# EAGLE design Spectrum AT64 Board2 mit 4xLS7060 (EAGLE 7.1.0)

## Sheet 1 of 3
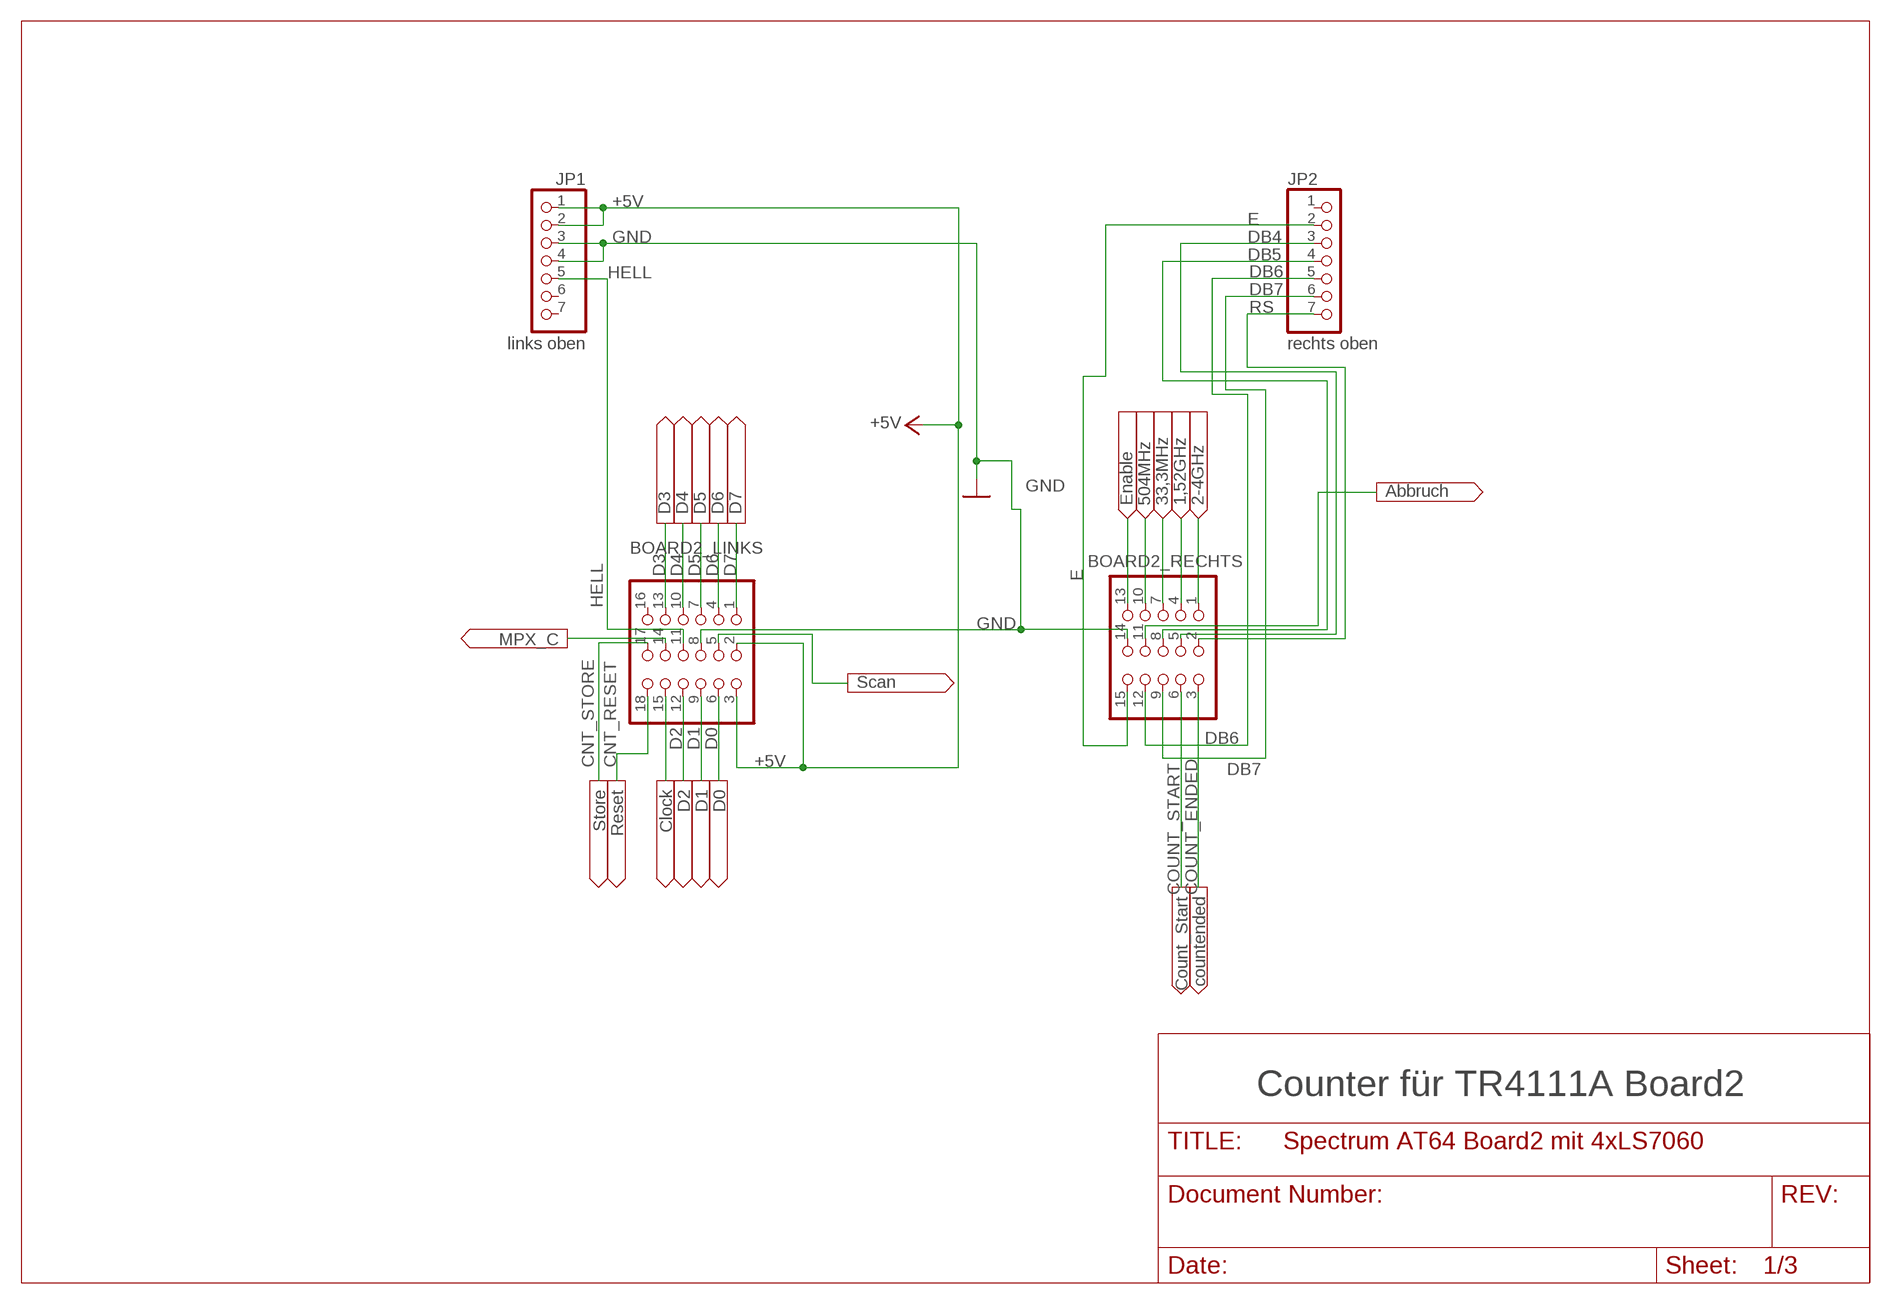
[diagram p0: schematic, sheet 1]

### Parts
BOARD2_LINKS  links  3X06  [3X06]
BOARD2_RECHTS  rechts  PINHEAD3X05  [3X05]
JP1  links oben  PINHD-1X7  [1X07]
JP2  rechts oben  PINHD-1X7  [1X07]

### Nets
1,52GHZ: BOARD2_RECHTS.4 ; also sheet 3
2-4GHZ: BOARD2_RECHTS.1 ; also sheet 3
33,3MHZ: BOARD2_RECHTS.7 ; also sheet 3
504MHZ: BOARD2_RECHTS.10 ; also sheet 3
+5V: BOARD2_LINKS.2 BOARD2_LINKS.3 JP1.1 JP1.2 ; also sheet 2,3
ABBRUCH: BOARD2_RECHTS.11 ; also sheet 2
CLOCK: BOARD2_LINKS.15 ; also sheet 2
CNT_RESET: BOARD2_LINKS.18 ; also sheet 3
CNT_STORE: BOARD2_LINKS.17 ; also sheet 3
COUNT_ENDED: BOARD2_RECHTS.3 ; also sheet 2
COUNT_START: BOARD2_RECHTS.6 ; also sheet 2
D0: BOARD2_LINKS.6 ; also sheet 3
D1: BOARD2_LINKS.9 ; also sheet 3
D2: BOARD2_LINKS.12 ; also sheet 3
D3: BOARD2_LINKS.13 ; also sheet 3
D4: BOARD2_LINKS.10 ; also sheet 3
D5: BOARD2_LINKS.7 ; also sheet 3
D6: BOARD2_LINKS.4 ; also sheet 3
D7: BOARD2_LINKS.1 ; also sheet 3
DB4: BOARD2_RECHTS.5 JP2.3
DB5: BOARD2_RECHTS.8 JP2.4
DB6: BOARD2_RECHTS.12 JP2.5
DB7: BOARD2_RECHTS.9 JP2.6
E: BOARD2_RECHTS.15 JP2.2
ENABLE: BOARD2_RECHTS.13 ; also sheet 3
GND: BOARD2_LINKS.8 BOARD2_RECHTS.14 JP1.3 JP1.4 ; also sheet 2,3
HELL: BOARD2_LINKS.11 JP1.5
MPX_C: BOARD2_LINKS.14 ; also sheet 2
RS: BOARD2_RECHTS.2 JP2.7
SCAN: BOARD2_LINKS.5 ; also sheet 3
Unconnected: BOARD2_LINKS.16 JP1.6 JP1.7 JP2.1

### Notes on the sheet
- Counter für TR4111A Board2

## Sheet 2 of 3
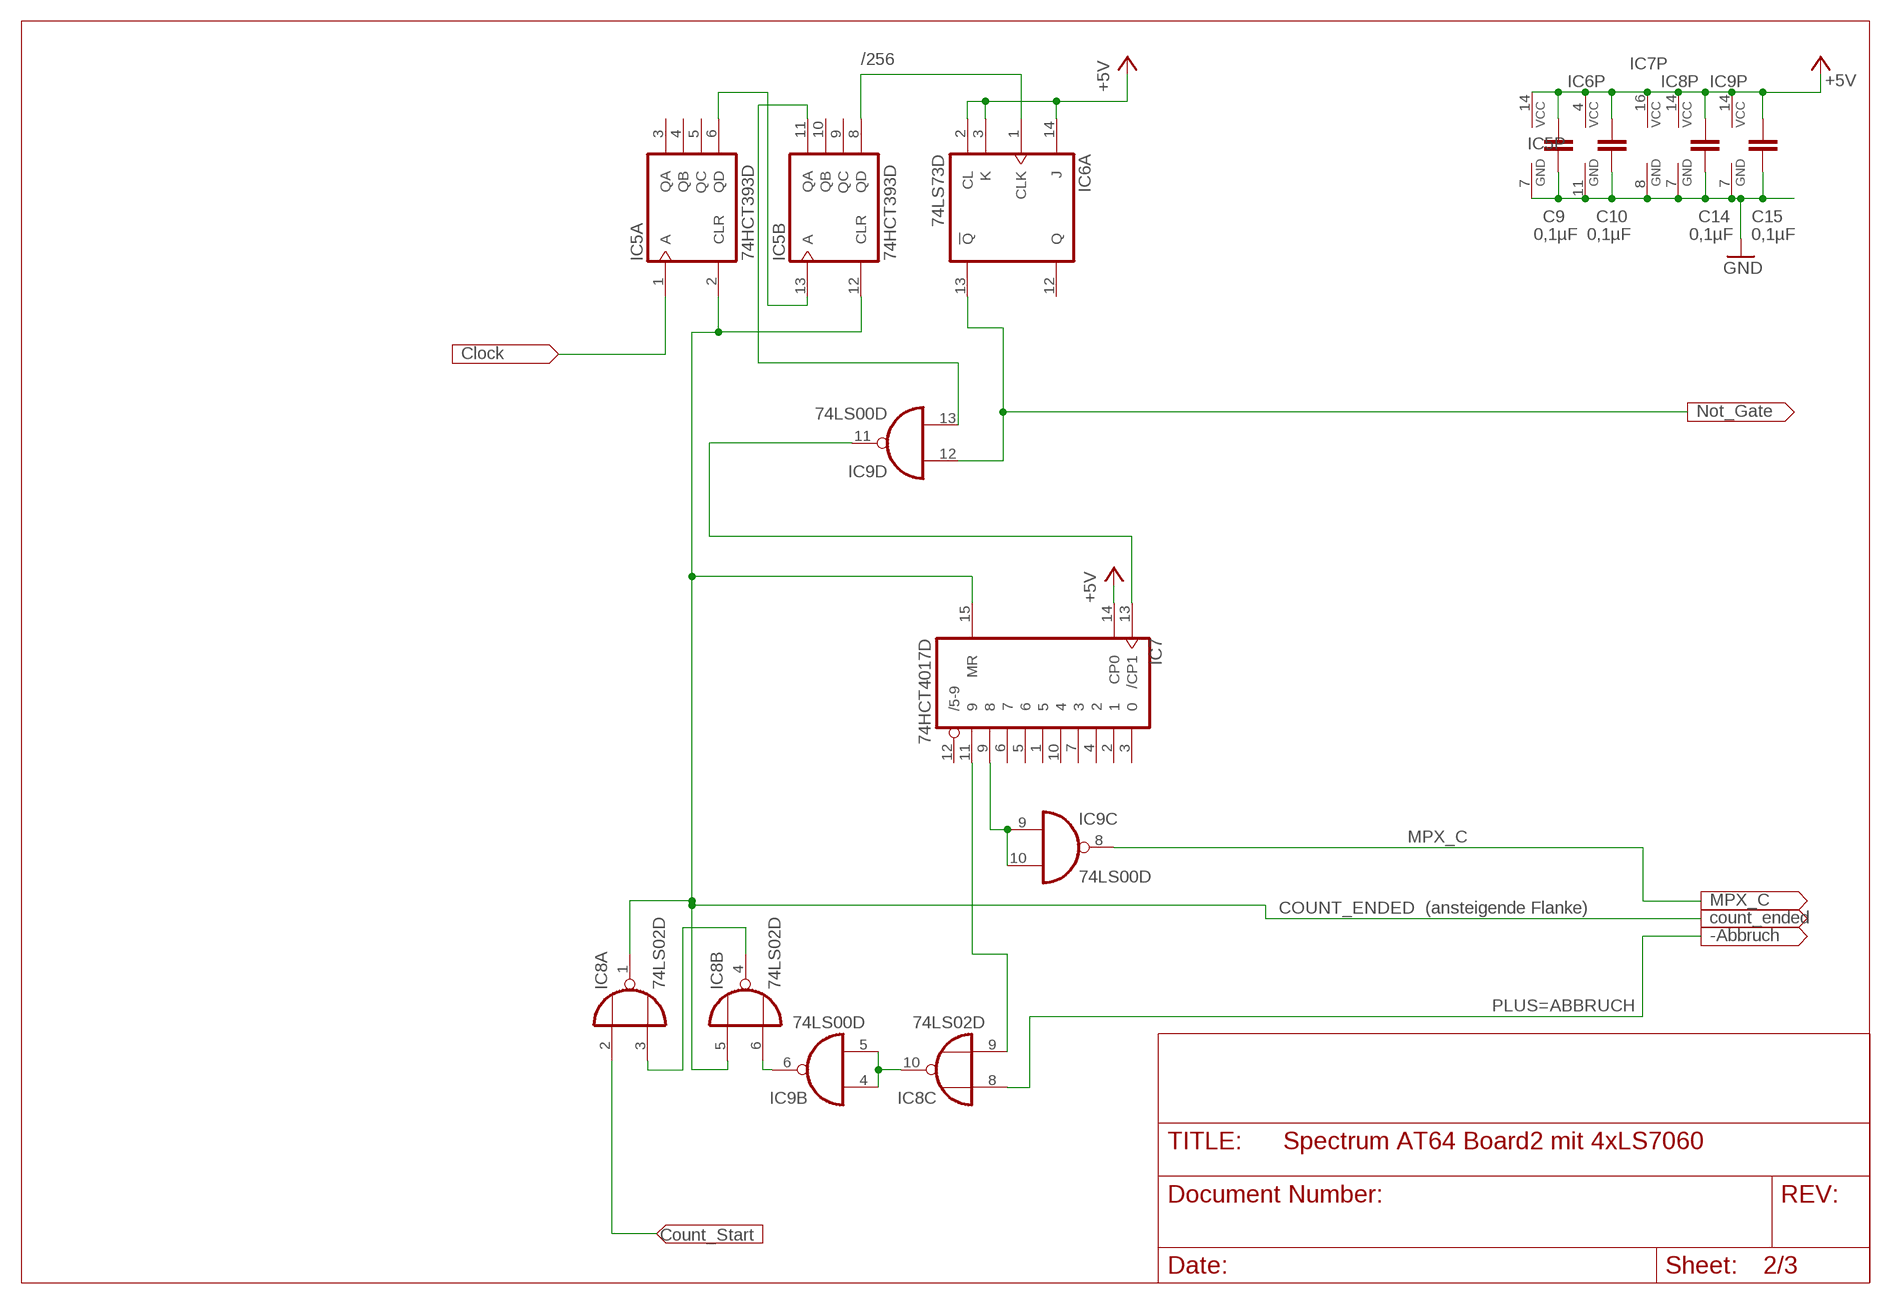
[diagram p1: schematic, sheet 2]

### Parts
C9  0,1µF  C-EUC0805  [C0805]
C10  0,1µF  C-EUC0805  [C0805]
C14  0,1µF  C-EUC0805  [C0805]
C15  0,1µF  C-EUC0805  [C0805]
IC5  74HCT393D  [SO14]
IC6  74LS73D  [SO14]
IC7  74HCT4017D  [SO16]
IC8  74LS02D  [SO14]
IC9  74LS00D  [SO14]

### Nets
+5V: C9.1 C10.1 C14.1 C15.1 IC5.14(P:VCC) IC6.2(A:CL) IC6.3(A:K) IC6.4(P:VCC) IC6.14(A:J) IC7.14(CP0) IC7.16(VCC) IC8.14(P:VCC) IC9.14(P:VCC) ; also sheet 1,3
ABBRUCH: IC8.8(C:I0) ; also sheet 1
CLOCK: IC5.1(A:A) ; also sheet 1
COUNT_ENDED: IC5.2(A:CLR) IC5.12(B:CLR) IC7.15(MR) IC8.1(A:O) IC8.5(B:I0) ; also sheet 1
COUNT_START: IC8.2(A:I0) ; also sheet 1
GND: C9.2 C10.2 C14.2 C15.2 IC5.7(P:GND) IC6.11(P:GND) IC7.8(GND) IC8.7(P:GND) IC9.7(P:GND) ; also sheet 1,3
MPX_C: IC9.8(C:O) ; also sheet 1
N$3: IC8.10(C:O) IC9.4(B:I0) IC9.5(B:I1)
N$4: IC7.11 IC8.9(C:I1)
N$8: IC7.9 IC9.9(C:I0) IC9.10(C:I1)
N$11: IC7.13(/CP1) IC9.11(D:O)
N$16: IC5.8(B:QD) IC6.1(A:CLK)
N$23: IC8.3(A:I1) IC8.4(B:O)
N$24: IC8.6(B:I1) IC9.6(B:O)
N$25: IC5.11(B:QA) IC9.13(D:I1)
NOT_GATE: IC6.13(A:!Q) IC9.12(D:I0) ; also sheet 3
OPEN: IC5.6(A:QD) IC5.13(B:A)
Unconnected: IC5.3(A:QA) IC5.4(A:QB) IC5.5(A:QC) IC5.9(B:QC) IC5.10(B:QB) IC6.5(B:CLK) IC6.6(B:CL) IC6.7(B:J) IC6.8(B:!Q) IC6.9(B:Q) IC6.10(B:K) IC6.12(A:Q) IC7.1 IC7.2 IC7.3 IC7.4 IC7.5 IC7.6 IC7.7 IC7.10 IC7.12(/5-9) IC8.11(D:I0) IC8.12(D:I1) IC8.13(D:O) IC9.1(A:I0) IC9.2(A:I1) IC9.3(A:O)

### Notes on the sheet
- /256
- (ansteigende Flanke)
- PLUS=

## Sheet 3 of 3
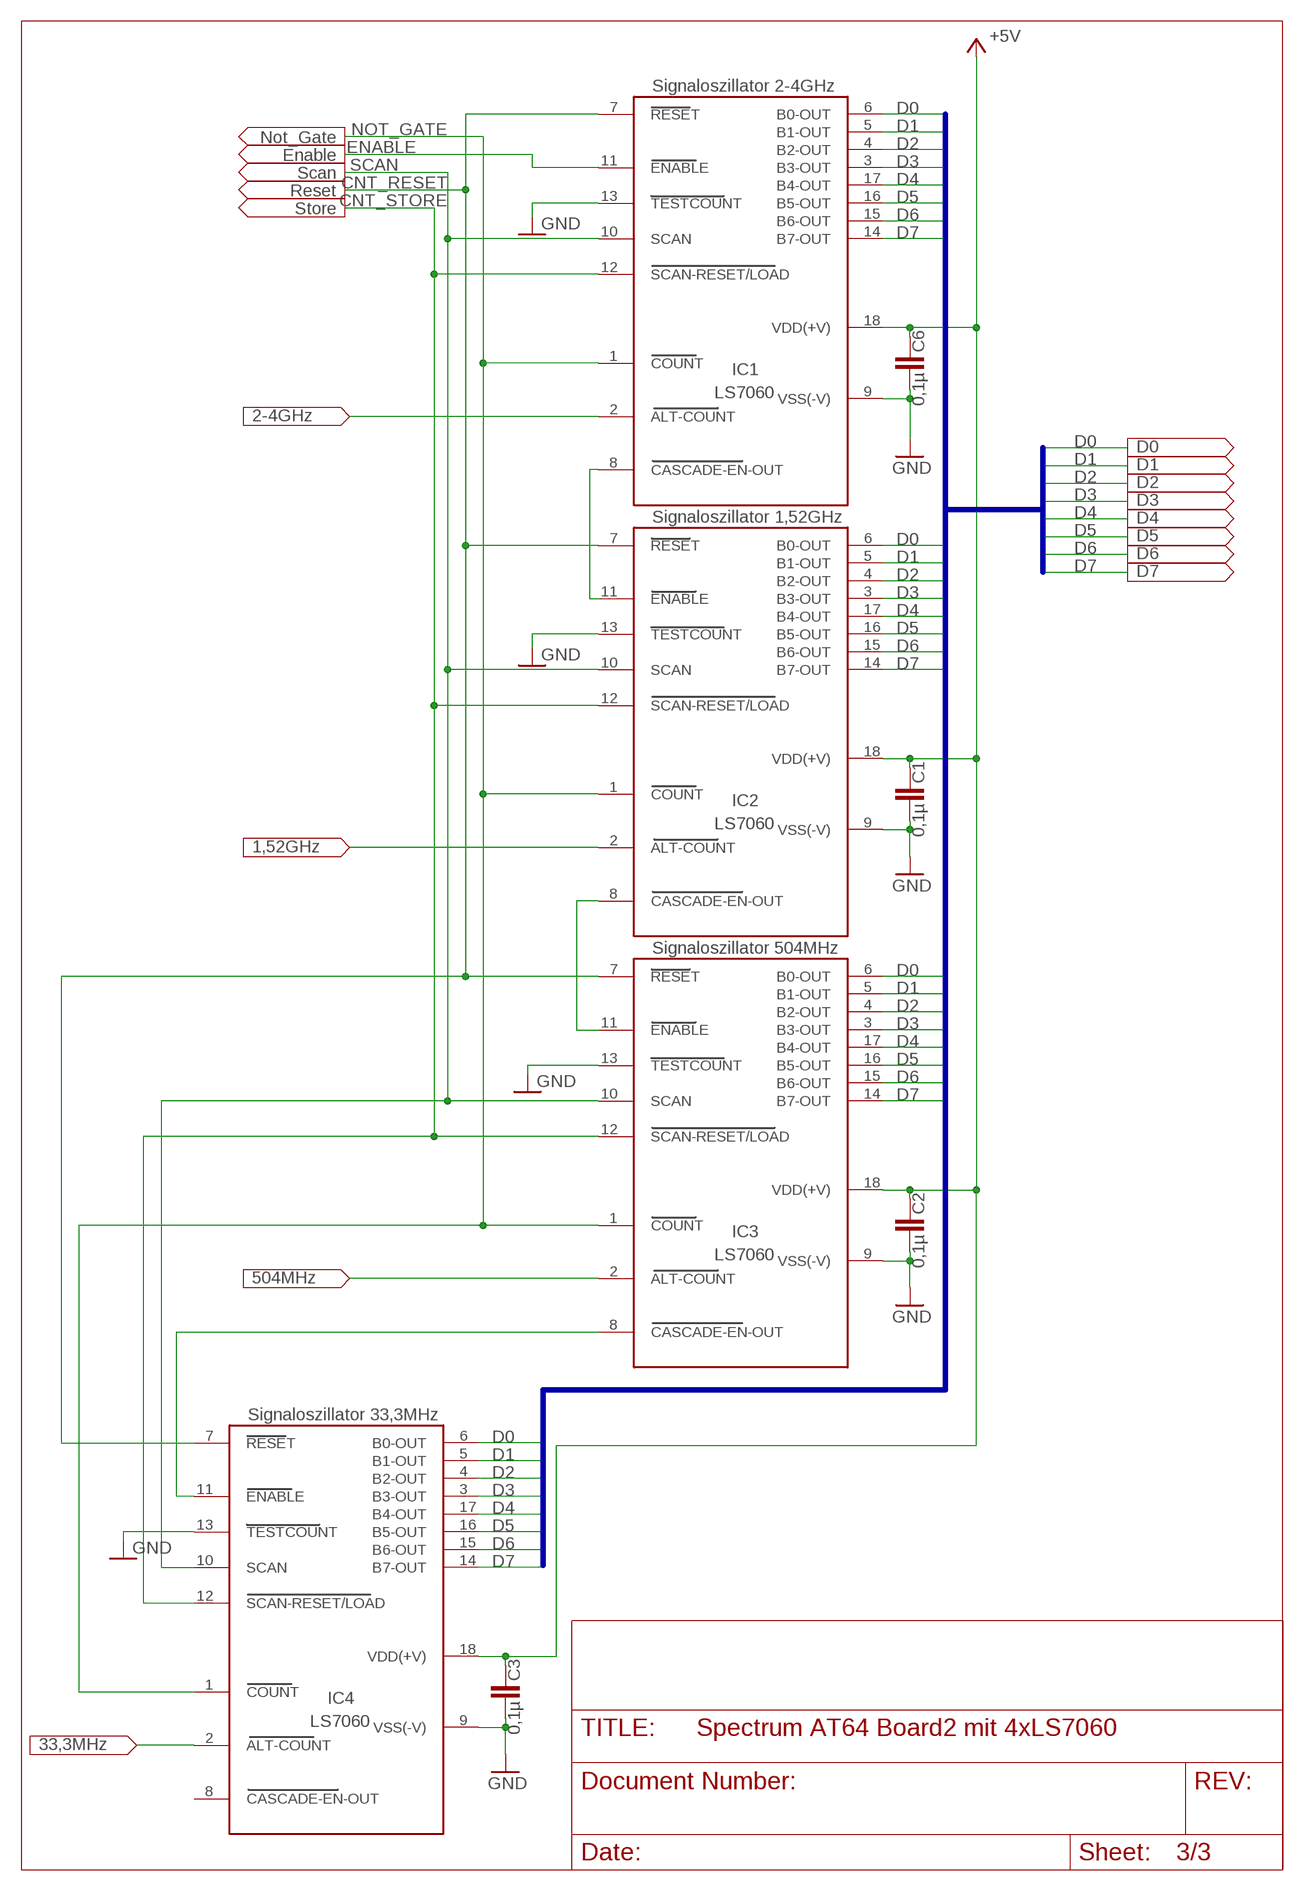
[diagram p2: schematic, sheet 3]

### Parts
C1  0,1µ  C-EU025-025X050  [C025-025X050]
C2  0,1µ  C-EU025-025X050  [C025-025X050]
C3  0,1µ  C-EU025-025X050  [C025-025X050]
C6  0,1µ  C-EU025-025X050  [C025-025X050]
IC1  LS7060  [DIL18]
IC2  LS7060  [DIL18]
IC3  LS7060  [DIL18]
IC4  LS7060  [DIL18]

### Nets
1,52GHZ: IC2.2(ALT-COUNT) ; also sheet 1
2-4GHZ: IC1.2(ALT-COUNT) ; also sheet 1
33,3MHZ: IC4.2(ALT-COUNT) ; also sheet 1
504MHZ: IC3.2(ALT-COUNT) ; also sheet 1
+5V: C1.1 C2.1 C3.1 C6.1 IC1.18(VDD(+V)) IC2.18(VDD(+V)) IC3.18(VDD(+V)) IC4.18(VDD(+V)) ; also sheet 1,2
CNT_RESET: IC1.7(RESET) IC2.7(RESET) IC3.7(RESET) IC4.7(RESET) ; also sheet 1
CNT_STORE: IC1.12(SCAN-RESET/LOAD) IC2.12(SCAN-RESET/LOAD) IC3.12(SCAN-RESET/LOAD) IC4.12(SCAN-RESET/LOAD) ; also sheet 1
D0: IC1.6(B0-OUT) IC2.6(B0-OUT) IC3.6(B0-OUT) IC4.6(B0-OUT) ; also sheet 1
D1: IC1.5(B1-OUT) IC2.5(B1-OUT) IC3.5(B1-OUT) IC4.5(B1-OUT) ; also sheet 1
D2: IC1.4(B2-OUT) IC2.4(B2-OUT) IC3.4(B2-OUT) IC4.4(B2-OUT) ; also sheet 1
D3: IC1.3(B3-OUT) IC2.3(B3-OUT) IC3.3(B3-OUT) IC4.3(B3-OUT) ; also sheet 1
D4: IC1.17(B4-OUT) IC2.17(B4-OUT) IC3.17(B4-OUT) IC4.17(B4-OUT) ; also sheet 1
D5: IC1.16(B5-OUT) IC2.16(B5-OUT) IC3.16(B5-OUT) IC4.16(B5-OUT) ; also sheet 1
D6: IC1.15(B6-OUT) IC2.15(B6-OUT) IC3.15(B6-OUT) IC4.15(B6-OUT) ; also sheet 1
D7: IC1.14(B7-OUT) IC2.14(B7-OUT) IC3.14(B7-OUT) IC4.14(B7-OUT) ; also sheet 1
ENABLE: IC1.11(ENABLE) ; also sheet 1
GND: C1.2 C2.2 C3.2 C6.2 IC1.9(VSS(-V)) IC1.13(TESTCOUNT) IC2.9(VSS(-V)) IC2.13(TESTCOUNT) IC3.9(VSS(-V)) IC3.13(TESTCOUNT) IC4.9(VSS(-V)) IC4.13(TESTCOUNT) ; also sheet 1,2
N$5: IC1.8(CASCADE-EN-OUT) IC2.11(ENABLE)
N$6: IC2.8(CASCADE-EN-OUT) IC3.11(ENABLE)
N$7: IC3.8(CASCADE-EN-OUT) IC4.11(ENABLE)
NOT_GATE: IC1.1(COUNT) IC2.1(COUNT) IC3.1(COUNT) IC4.1(COUNT) ; also sheet 2
SCAN: IC1.10(SCAN) IC2.10(SCAN) IC3.10(SCAN) IC4.10(SCAN) ; also sheet 1
Unconnected: IC4.8(CASCADE-EN-OUT)

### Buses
D[0..7]

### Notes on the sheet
- Signaloszillator 2-4GHz
- Signaloszillator 1,52GHz
- Signaloszillator 504MHz
- Signaloszillator 33,3MHz

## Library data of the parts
BOARD2_LINKS = 1Eigene:3X06
BOARD2_RECHTS = 1Eigene:PINHEAD3X05
C1-C3 C6 C9 C10 C14 C15 = rcl:C-EU: CAPACITOR, European symbol
IC1-IC4 = 1Eigene:LS7060
IC5 = 74xx-eu:74*393: Dual 4-bit decade and binary COUNTER
IC6 = 74xx-eu:74*73: Dual J-K FLIP FLOP, clear
IC7 = 1Eigene:74HCT4017D
IC8 = 74xx-eu:74*02: Quad 2-input NOR gate
IC9 = 74xx-eu:74*00: Quad 2-input NAND gate
JP1 JP2 = pinhead:PINHD-1X7: PIN HEADER

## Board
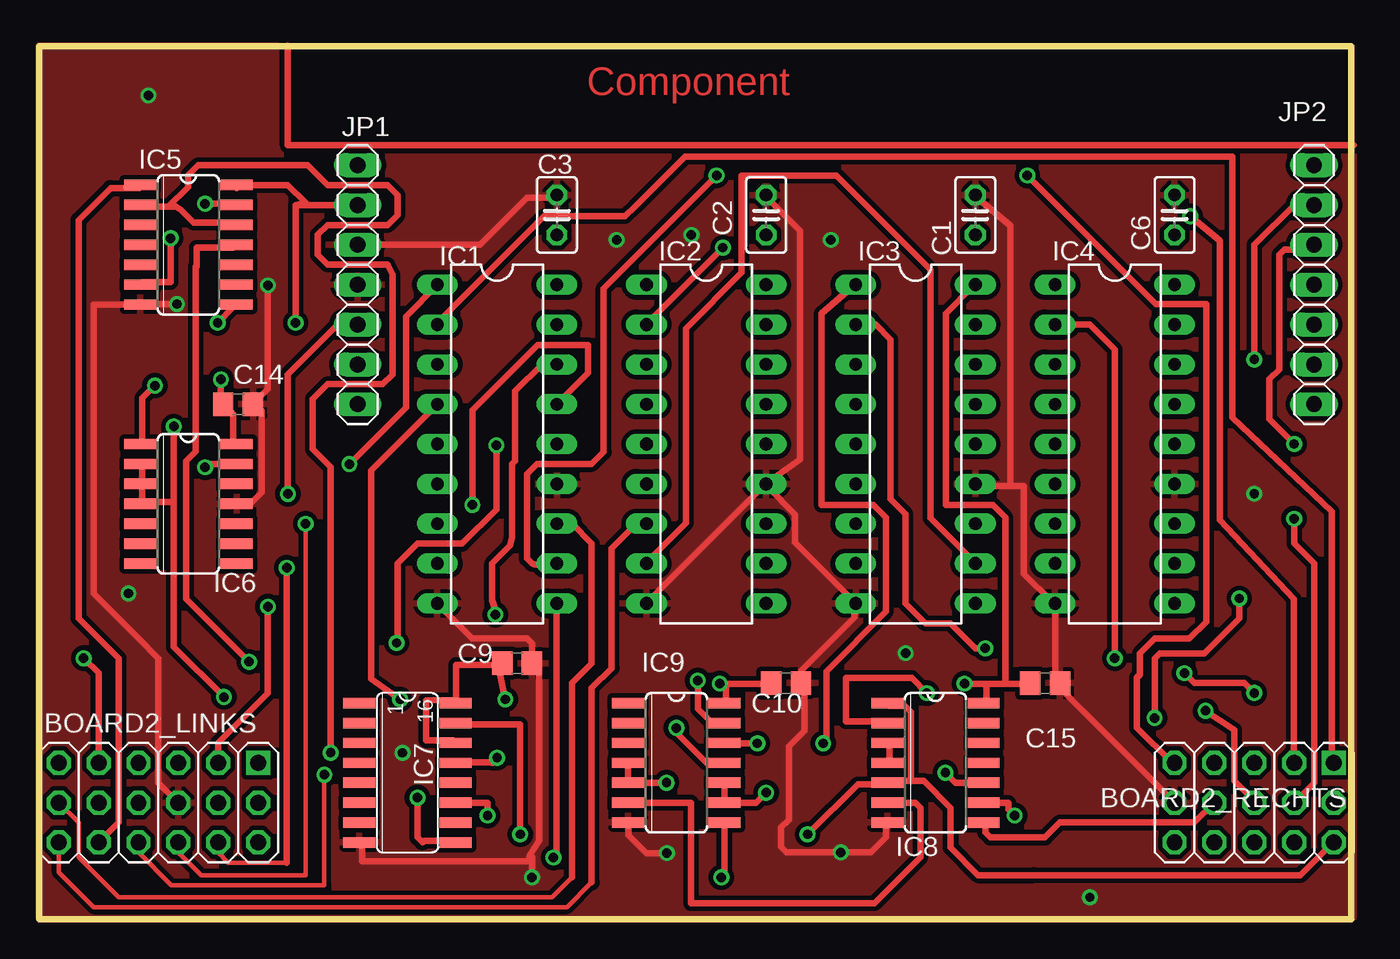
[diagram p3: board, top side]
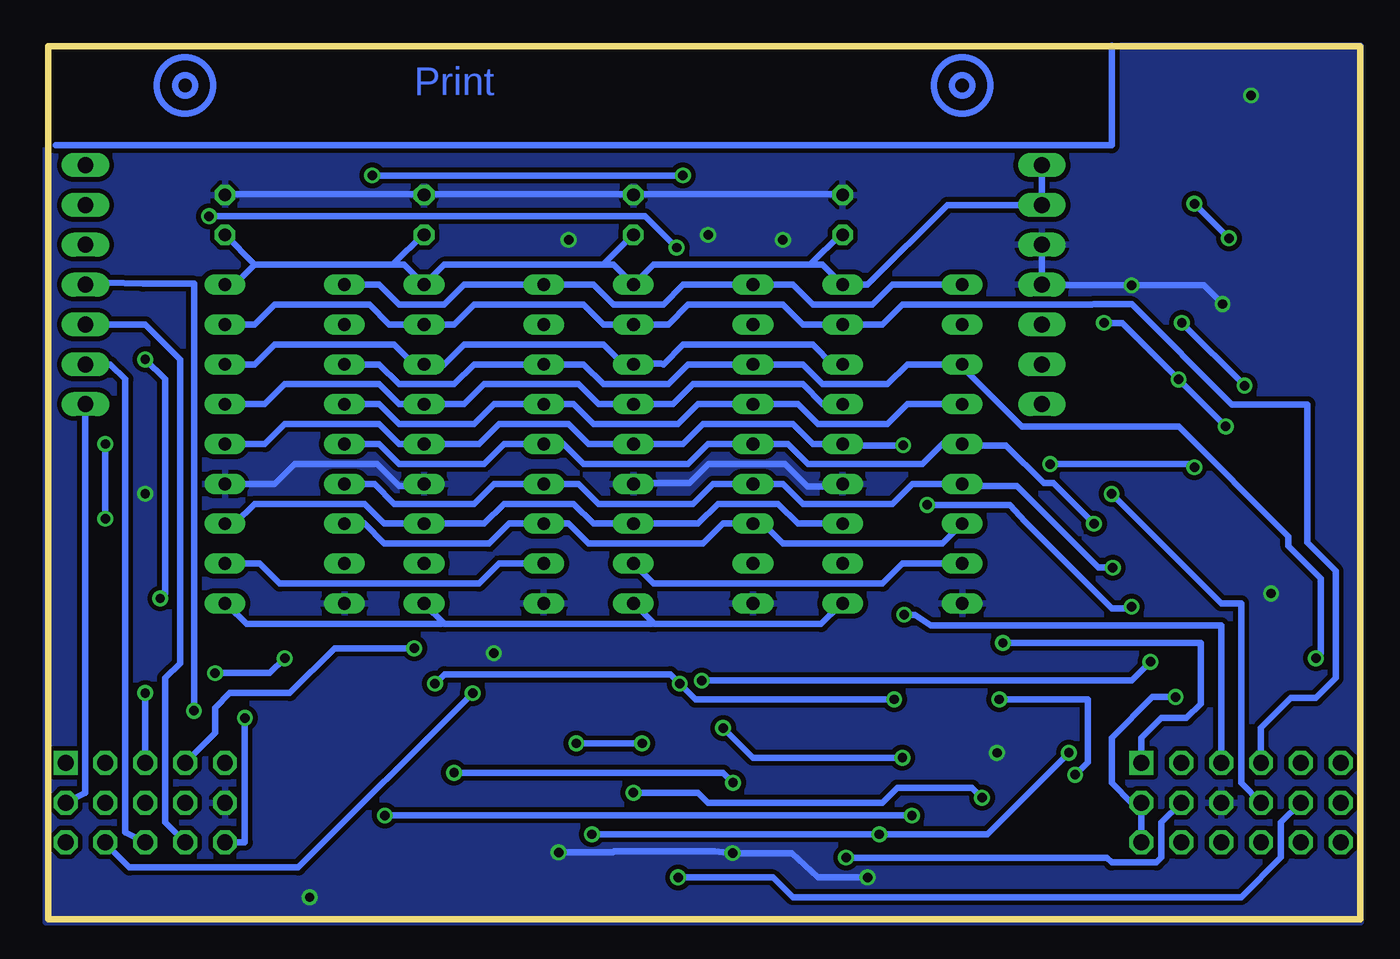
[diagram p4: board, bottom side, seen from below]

Size 83.63 x 55.66 mm. Coordinates in mm from the lower left corner, seen from the top.
Outline: 0,0 83.63,0 83.63,55.66 0,55.66 0,0
Copper layers (1*16): Top 0.035mm / dielectric 1.5mm / Bottom 0.035mm
Design rules "default *": minimum track width 0.4mm, minimum drill 0.6mm, track to track 0.3mm, track to pad 0.3mm, pad to pad 0.3mm, via to via 0.3mm, smd to smd 0.3mm, copper to edge 0mil, drill to drill 0.4mm, minimum pad ring 10mil, minimum via ring 8mil, stop-mask expansion 4mil, vias tented up to drill 0mil, thermal gap 10mil

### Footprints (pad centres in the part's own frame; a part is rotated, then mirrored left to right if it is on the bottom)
3X06 = drill 1.016 square: 1 6.35,2.54 | drill 1.016 octagon: 2 6.35,0; 3 6.35,-2.54; 4 3.81,2.54; 5 3.81,0; 6 3.81,-2.54; 7 1.27,2.54; 8 1.27,0; 9 1.27,-2.54; 10 -1.27,2.54; 11 -1.27,0; 12 -1.27,-2.54; 13 -3.81,2.54; 14 -3.81,0; 15 -3.81,-2.54; 16 -6.35,2.54; 17 -6.35,0; 18 -6.35,-2.54
3X05 = drill 1.016 square: 1 5.08,2.54 | drill 1.016 octagon: 2 5.08,0; 3 5.08,-2.54; 4 2.54,2.54; 5 2.54,0; 6 2.54,-2.54; 7 0,2.54; 8 0,0; 9 0,-2.54; 10 -2.54,2.54; 11 -2.54,0; 12 -2.54,-2.54; 13 -5.08,2.54; 14 -5.08,0; 15 -5.08,-2.54
C025-025X050 = drill 0.813 octagon: 1 -1.27,0; 2 1.27,0
C0805 = smd 1.3 x 1.5: 1 -0.95,0; 2 0.95,0
DIL18 = drill 0.813 long: 1 -10.16,-3.81; 2 -7.62,-3.81; 3 -5.08,-3.81; 4 -2.54,-3.81; 5 0,-3.81; 6 2.54,-3.81; 7 5.08,-3.81; 8 7.62,-3.81; 9 10.16,-3.81; 10 10.16,3.81; 11 7.62,3.81; 12 5.08,3.81; 13 2.54,3.81; 14 0,3.81; 15 -2.54,3.81; 16 -5.08,3.81; 17 -7.62,3.81; 18 -10.16,3.81
SO14 = smd 0.66 x 2.032: 1 -3.81,-3.073; 2 -2.54,-3.073; 3 -1.27,-3.073; 4 0,-3.073; 5 1.27,-3.073; 6 2.54,-3.073; 7 3.81,-3.073; 8 3.81,3.073; 9 2.54,3.073; 10 1.27,3.073; 11 0,3.073; 12 -1.27,3.073; 13 -2.54,3.073; 14 -3.81,3.073
SO16 = smd 0.66 x 2.032: 1 -4.445,-3.073; 2 -3.175,-3.073; 3 -1.905,-3.073; 4 -0.635,-3.073; 5 0.635,-3.073; 6 1.905,-3.073; 7 3.175,-3.073; 8 4.445,-3.073; 9 4.445,3.073; 10 3.175,3.073; 11 1.905,3.073; 12 0.635,3.073; 13 -0.635,3.073; 14 -1.905,3.073; 15 -3.175,3.073; 16 -4.445,3.073
1X07 = drill 1.016 long: 1 -7.62,0; 2 -5.08,0; 3 -2.54,0; 4 0,0; 5 2.54,0; 6 5.08,0; 7 7.62,0

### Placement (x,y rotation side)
BOARD2_LINKS  7.59,7.44 0 top
BOARD2_RECHTS  77.44,7.44 0 top
C1  59.66,44.91 90 top
C2  46.33,44.91 90 top
C3  32.99,44.91 90 top
C6  72.36,44.91 90 top
C9  30.45,16.33 0 top
C10  47.6,15.06 0 top
C14  12.67,32.84 0 top
C15  64.11,15.06 0 top
IC1  29.18,30.3 270 top
IC2  42.52,30.3 270 top
IC3  55.85,30.3 270 top
IC4  68.55,30.3 270 top
IC5  9.5,43 270 top
IC6  9.5,26.49 270 top
IC7  23.47,9.35 270 top
IC8  57.12,9.98 270 top
IC9  40.61,9.98 270 top
JP1  20.29,40.46 270 top
JP2  81.25,40.46 270 top

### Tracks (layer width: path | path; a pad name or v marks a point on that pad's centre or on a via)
1,52GHZ  (via drill 0.6)
  Top 0.4: v43.57,42.82 38.77,38.02 IC2.2 | v73.37,44.82 75.26,43.26 75.26,25.46 79.97,20.42 79.97,10.02 BOARD2_RECHTS.4
  Bottom 0.4: v43.57,42.82 45.57,44.82 v73.37,44.82
2-4GHZ
  Top 0.4: IC1.2 25.37,38.02 32.17,44.82 37.34,44.82 37.97,45.42 41.17,48.62 76.06,48.62 76.06,32.01 82.37,26.01 82.37,10.02 BOARD2_RECHTS.1
33,3MHZ  (via drill 0.6 pad 1.02)
  Top 0.4: v77.44,14.43 76.81,15.06 73.63,15.06 v73,15.7 | v68.55,16.65 68.55,36.34 66.97,37.92 IC4.2
  Bottom 0.4: v77.44,14.43 BOARD2_RECHTS.7 | v73,15.7 69.51,15.7 v68.55,16.65
504MHZ  (via drill 0.6 pad 1.02)
  Top 0.4: IC3.2 53.31,37.92 54.27,36.97 54.27,26.81 55.22,25.86 55.22,20.14 56.49,18.87 58.08,18.87 59.66,17.28 v60.3,17.28
  Bottom 0.4: v60.3,17.28 65.38,17.28 68.24,14.43 72.05,14.43 73,13.47 73,11.89 BOARD2_RECHTS.10
+5V  (via drill 0.6)
  Top 0.4: IC6.14 12.37,30.42 12.37,32.22 11.77,32.82 C14.1 11.57,33.02 v11.57,34.42 | IC6.2 6.57,29.02 6.57,27.82 IC6.3 6.57,27.62 6.57,26.62 IC6.4 6.77,26.62 8.57,26.62 | 8.57,26.62 8.57,17.37 v11.77,14.17 | 8.57,26.62 v8.57,31.42 | 43.77,15.02 46.57,15.02 C10.1 | 43.77,15.02 43.77,13.82 IC9.14 | 26.57,13.99 26.57,16.22 29.37,16.22 C9.1 29.37,16.02 29.37,15.62 v29.7,14.02 | 26.57,13.99 26.57,13.82 IC7.16 | v43.37,15.02 43.77,15.02 | 61.57,15.02 60.37,15.02 | 61.57,15.02 62.97,15.02 C15.1 | 60.37,15.02 60.37,13.82 IC8.14 | 12.57,46.62 IC5.14 15.85,46.81 16.97,45.69 16.34,45.54 | 20.17,45.62 JP1.2 16.34,45.54 | 61.57,15.02 61.57,25.62 60.77,26.42 57.77,26.42 57.77,38.62 59.57,40.42 IC3.18 | 60.37,15.02 v58.97,15.02 | v16.34,38.02 16.34,45.54 | 26.57,13.99 24.66,13.97 24.66,11.42 26.37,11.42 IC7.14
  Bottom 0.4: IC4.18 71.73,40.46 70.46,41.73 | 61.57,41.73 60.93,41.73 IC3.18 58.39,41.73 48.17,41.73 | 61.57,41.73 70.46,41.73 | 48.17,41.73 47.6,41.73 IC2.18 45.06,41.73 34.97,41.73 | 34.97,41.73 34.26,41.73 IC1.18 31.41,40.46 26.33,45.54 JP1.2 JP1.1 | v8.57,31.42 v11.57,34.42 15.17,38.02 v16.34,38.02 | v29.7,14.02 42.37,14.02 v43.37,15.02 43.97,15.62 58.37,15.62 v58.97,15.02 | C3.1 33.17,43.62 34.97,41.82 34.97,41.73 | C2.1 46.37,43.62 48.17,41.82 48.17,41.73 | C1.1 59.77,43.62 61.57,41.82 61.57,41.73 | 70.46,41.73 C6.1
  Bottom 0.406: v11.77,14.17 13.24,14.17 15.85,11.57 15.85,8.71 14.58,7.44 BOARD2_LINKS.2 BOARD2_LINKS.3
ABBRUCH
  Top 0.406: BOARD2_RECHTS.11 73.63,6.17 65.06,6.17 64.11,5.22 60.62,5.22 60.3,5.54 60.3,6.07 IC8.8
CLOCK
  Top 0.4: 6.37,46.62 IC5.1
  Top 0.406: 6.37,46.62 4.55,46.62 2.51,44.59 2.51,19.19 5.05,16.65 5.05,6.17 BOARD2_LINKS.15
CNT_RESET
  Top 0.3: 35.22,2.36 33.63,0.78 3.47,0.78 1.24,3 BOARD2_LINKS.18
  Top 0.406: IC2.7 38.07,25.22 36.49,23.63 36.49,16.01 35.22,14.74 35.22,2.36
  Bottom 0.4: IC4.7 63.47,25.22 62.2,23.95 55.54,23.95 54.27,25.22 IC3.7 50.46,25.22 49.19,23.95 41.88,23.95 40.61,25.22 IC2.7
  Bottom 0.406: IC2.7 38.07,25.22 36.8,23.95 26.64,23.95 IC1.7
CNT_STORE
  Top 0.3: 33.95,2.68 32.68,1.41 5.05,1.41 2.51,3.95 2.51,6.17 BOARD2_LINKS.17
  Top 0.406: 33.95,2.68 33.95,15.06 35.22,16.33 35.22,23.95 33.95,25.22 IC1.12
  Bottom 0.4: 46.17,25.22 IC2.12 48.87,25.22 50.14,26.49 54.58,26.49 55.85,25.22 IC3.12 62.2,25.22 63.47,26.49 70.46,26.49 71.73,25.22 IC4.12
  Bottom 0.406: 46.17,25.22 42.2,25.22 40.93,26.49 37.12,26.49 35.85,25.22 IC1.12
COUNT_ENDED  (via drill 0.6)
  Top 0.4: 63.37,2.82 80.37,2.82 82.37,4.82 BOARD2_RECHTS.3 | 8.23,45.42 6.57,45.42 IC5.2 | 8.23,45.42 8.74,45.42 9.06,45.22 9.86,44.42 12.37,44.42 IC5.12 12.77,44.22 | 55.57,8.82 54.17,8.82 IC8.5 53.97,8.62 52.17,8.62 v48.97,5.42 | 55.57,8.82 55.57,13.22 55.17,13.62 54.17,13.62 IC8.1 | v30.66,5.42 30.66,12.42 26.57,12.42 IC7.15 | 8.23,45.42 9.5,46.69 9.5,47.45 10.13,48.08 17.12,48.08 18.39,46.81 22.2,46.81 22.83,46.18 22.83,44.91 22.2,44.27 18.39,44.27 17.75,43.64 17.75,42.37 18.39,41.73 22.2,41.73 22.52,41.1 22.52,34.75 21.88,34.11 18.39,34.11 17.44,33.16 17.44,29.99 18.57,28.85 v18.57,10.62 | 55.57,8.82 56.38,8.82 58.08,7.13 58.08,6.32
  Top 0.406: 63.37,2.82 59.84,2.82 58.08,4.59 58.08,6.32
  Bottom 0.4: v48.97,5.42 v30.66,5.42 23.77,5.42 v18.57,10.62
COUNT_START  (via drill 0.6)
  Top 0.4: IC8.2 53.97,12.62 51.41,12.62 51.41,15.38 55.62,15.38 v56.57,14.42
  Bottom 0.4: v56.57,14.42 67.69,3.3 78.46,3.3 79.97,4.82 BOARD2_RECHTS.6
D0  (via drill 0.6)
  Top 0.3: 15.77,3.62 12.05,3.62 11.4,4.27 BOARD2_LINKS.6
  Top 0.4: 15.77,3.62 v15.77,22.42
  Bottom 0.4: IC4.6 62.84,27.76 61.57,26.49 56.49,26.49 55.22,27.76 IC3.6 49.82,27.76 48.55,26.49 42.52,26.49 41.25,27.76 IC2.6 36.8,27.76 35.53,26.49 29.82,26.49 28.55,27.76 IC1.6 25.37,27.62 21.88,27.62
  Bottom 0.406: v15.77,22.42 16.68,22.42 21.88,27.62
D1  (via drill 0.6)
  Top 0.3: v16.97,25.22 16.97,2.82 10.31,2.82 8.86,4.27 BOARD2_LINKS.9
  Bottom 0.4: IC4.5 62.52,30.3 61.25,29.03 55.85,29.03 54.58,30.3 IC3.5 50.77,30.3 49.5,29.03 42.84,29.03 41.57,30.3 IC2.5 36.49,30.3 35.22,29.03 27.91,29.03 26.64,30.3 IC1.5 25.37,30.22 22.57,30.22 20.17,27.82 19.57,27.82 v16.97,25.22
D2  (via drill 0.6)
  Top 0.3: v18.17,9.22 18.17,2.18 8.42,2.18 6.32,4.27 BOARD2_LINKS.12
  Top 0.4: v23.01,14.02 21.15,15.34 21.15,28.6 25.37,32.82 IC1.4
  Bottom 0.4: IC4.4 62.52,32.84 61.25,31.57 56.49,31.57 55.22,32.84 IC3.4 50.14,32.84 48.87,31.57 43.47,31.57 42.2,32.84 IC2.4 35.85,32.84 34.58,31.57 30.14,31.57 28.87,32.84 IC1.4 | v18.17,9.22 17.37,10.02 17.37,14.02 v23.01,14.02
D3  (via drill 0.6 pad 1.02)
  Top 0.406: v2.83,16.65 3.78,15.7 BOARD2_LINKS.13
  Bottom 0.4: IC4.3 62.52,35.38 61.25,34.11 57.76,34.11 56.49,35.38 IC3.3 49.5,35.38 48.23,34.11 44.11,34.11 42.84,35.38 IC2.3 35.53,35.38 34.26,34.11 30.14,34.11 28.87,35.38 IC1.3 25.37,35.22 21.57,31.42 11.57,31.42 4.57,24.42 4.57,23.79 2.51,21.73 2.51,16.97 v2.83,16.65
D4
  Bottom 0.4: IC4.17 70.46,37.92 69.19,39.19 63.16,39.19 61.89,37.92 IC3.17 57.76,37.92 56.49,39.19 49.5,39.19 48.23,37.92 IC2.17 44.11,37.92 42.84,39.19 36.8,39.19 35.53,37.92 IC1.17 30.45,37.92 29.18,39.19 17.12,39.19 16.97,39.22 14.57,39.22 8.17,32.82 3.37,32.82 3.37,24.02 1.56,22.21
  Bottom 0.406: 1.56,22.21 1.56,15.38 2.83,14.11 4.42,14.11 6.32,12.21 BOARD2_LINKS.10
D5  (via drill 0.6)
  Top 0.4: IC1.16 32.97,35.22
  Top 0.406: IC1.16 32.04,35.38 30.34,33.68 30.34,29.24 30.14,29.03 30.14,24.36 30.02,23.84 28.87,22.68 28.87,20.37 29.18,19.42 v29.07,19.42
  Bottom 0.4: IC4.16 70.46,35.38 69.19,36.65 61.57,36.65 60.3,35.38 IC3.16 58.39,35.38 57.12,36.65 48.23,36.65 46.96,35.38 46.77,35.42 46.37,35.42 IC2.16 46.17,35.42 44.57,35.42 44.42,35.38 43.15,36.65 34.9,36.65 33.63,35.38 33.57,35.42 33.17,35.42 IC1.16 | 8.86,18.74 27.37,18.74 28.37,19.42 v29.07,19.42
  Bottom 0.406: BOARD2_LINKS.7 8.86,18.74
D6  (via drill 0.6)
  Top 0.4: 14.57,14.42 v14.57,19.94 | v27.61,26.42 27.62,27.71 27.62,32.47 31.77,36.62 34.97,36.62 34.97,34.82 IC1.15
  Top 0.406: 14.57,14.42 11.4,11.25 BOARD2_LINKS.4
  Bottom 0.4: IC4.15 69.82,32.84 68.55,34.11 62.52,34.11 61.25,32.84 IC3.15 57.12,32.84 55.85,34.11 49.82,34.11 48.55,32.84 IC2.15 43.79,32.84 42.52,34.11 35.53,34.11 34.26,32.84 IC1.15 | 22.33,26.42 v27.61,26.42
  Bottom 0.406: 22.33,26.42 21.37,25.35 15.85,19.83 14.69,19.83 v14.57,19.94
D7  (via drill 0.6)
  Top 0.406: v29.14,30.22 29.14,26.13 26.96,23.95 24.1,23.95 22.83,22.68 22.83,17.68 v22.78,17.62
  Bottom 0.4: IC4.14 69.82,30.3 68.55,31.57 62.52,31.57 61.25,30.3 IC3.14 56.17,30.3 54.9,31.57 50.46,31.57 49.19,30.3 IC2.14 43.15,30.3 41.88,31.57 36.17,31.57 34.9,30.3 IC1.14 32.97,30.22 v29.14,30.22 | 10.17,17.62 v22.78,17.62
  Bottom 0.406: 10.17,17.62 10.17,13.75 11.09,12.84 12.67,12.84 13.94,11.57 BOARD2_LINKS.1
DB4  (via drill 0.6 pad 1.02)
  Top 0.4: BOARD2_RECHTS.5 81.25,8.71 81.25,22.68 79.98,23.95 v79.98,25.54 | v79.98,30.3 78.4,31.89 78.4,34.43 79.03,35.06 79.03,42.37 79.35,42.68 80.94,42.68 JP2.3
  Bottom 0.4: v79.98,25.54 v79.98,30.3
DB5  (via drill 0.6)
  Top 0.4: v74.34,13.3 76.17,12.1 76.17,8.82 77.37,7.62 BOARD2_RECHTS.8
  Bottom 0.4: v74.34,13.3 74.34,40.52 77.57,40.52 81.17,40.62 JP2.4
DB6
  Bottom 0.4: BOARD2_RECHTS.12 76.17,6.17 76.17,15.38 75.22,16.33 75.22,35.7 77.44,37.92 JP2.5
DB7
  Bottom 0.4: BOARD2_RECHTS.9 78.71,5.54 78.71,34.43 79.67,35.38 JP2.6
E  (via drill 0.6, 0.6 pad 1.02)
  Top 0.4: v77.44,35.7 77.44,43 79.98,45.54 JP2.2 | v76.49,20.46 76.49,19.19 74.27,16.97 71.41,16.97 71.09,16.65 v71.09,12.84
  Bottom 0.4: BOARD2_RECHTS.15 71.09,4.9 v71.09,12.84 | v76.49,20.46 76.17,20.78 76.17,34.43 v77.44,35.7
ENABLE  (via drill 0.6)
  Top 0.4: 33.17,22.82 IC1.11 32.97,22.62 31.57,22.62 31.41,22.68 | 35.97,40.22 v43.17,47.42 | v62.97,47.42 71.17,39.22 74.37,39.22 74.37,18.98 73.32,17.92 71.09,17.92 70.14,16.97 70.14,15.59 69.97,15.42 69.97,12.22 72.17,10.02 BOARD2_RECHTS.13
  Top 0.406: 35.97,40.22 35.97,29.79 35.22,29.03 31.72,29.03 31.09,28.4 31.09,23 31.41,22.68
  Bottom 0.4: v43.17,47.42 v62.97,47.42
GND  (via drill 0.6, 0.6 pad 0.81)
  Top 0.4: 31.27,4.12 31.17,3.7 20.57,3.7 20.57,4.82 IC7.8 | 31.27,4.12 31.86,5.02 31.86,15.62 31.57,16.22 C9.2 | 37.37,6.02 IC9.7 37.57,6.02 | 31.37,4.02 31.27,4.12 | IC8.7 53.97,6.02 53.97,5.25 53,4.27 v51.09,4.27 47.63,4.27 47.28,4.62 47.28,5.85 47.77,6.35 47.77,11.02 48.77,12.02 48.77,15.22 C10.2 48.57,15.86 51.97,19.26 51.97,20.02 IC3.9 51.97,20.22 48.17,24.02 48.17,25.82 46.37,27.62 IC2.13 | IC2.9 38.77,20.22 46.17,27.62 IC2.13 | IC4.9 64.77,20.02 64.77,15.42 64.97,15.22 C15.2 65.17,15.02 65.17,14.62 72.17,7.62 BOARD2_RECHTS.14 | 61.89,27.62 62.77,27.62 62.77,22.02 64.57,20.22 IC4.9 | 61.89,27.62 59.77,27.62 IC3.13 | IC4.9 64.77,20.22 | IC6.11 12.57,26.62 13.57,26.62 14.17,27.22 14.17,32.42 13.77,32.82 C14.2 13.77,33.02 14.57,33.82 v14.57,40.42 | v8.77,39.22 6.57,39.22 IC5.7 3.47,39.19 3.47,20.78 6.32,17.92 | JP1.3 20.37,43.02 28.1,43.02 31.1,46.02 32.97,46.02 C3.2 | 61.89,27.62 61.89,44.22 59.77,46.02 C1.2 | IC2.13 46.37,27.82 48.49,29.31 48.49,43.91 46.37,46.02 C2.2
  Top 0.406: 6.32,17.92 7.59,16.65 7.59,8.71 BOARD2_LINKS.8 | v31.41,2.68 31.41,3.99 31.37,4.02 | IC1.9 27.6,17.92 31.09,17.92 31.41,17.6 C9.2 | 37.57,6.02 37.57,5.36 38.71,4.22 v40.01,4.22
  Bottom 0.4: JP1.3 JP1.4 20.17,40.42 v14.57,40.42 9.97,40.42 v8.77,39.22 | IC1.13 33.17,27.82 32.94,27.59 35.22,27.59 36.66,29.02 41.54,29.02 42.74,27.82 46.17,27.82 IC2.13 | v40.01,4.22 41.17,4.33 47.57,4.33 47.63,4.27 v51.09,4.27 | C6.2 72.17,46.22 59.77,46.22 C1.2 59.57,46.22 46.37,46.22 C2.2 46.17,46.22 33.17,46.22 C3.2 | IC4.13 69.19,27.76 67.92,29.03 62.66,29.03 61.25,27.62 59.8,27.62 IC3.13
  Bottom 0.406: v40.01,4.22 36.21,4.22 34.58,2.68 v31.41,2.68
  other vias: 6.96,52.53 36.8,43.32 41.57,43.64 50.46,43.32 77.44,27.13 5.69,20.78 23.15,10.62 55.22,16.97 66.97,1.41
  pour Bottom (isolate 0.305): -0.03,55.7 15.85,55.7 15.85,49.35 83.79,49.35 83.79,-0.18 -0.03,-0.18
  pour Top: -0.03,55.7 15.85,55.7 15.85,49.35 83.79,49.35 83.79,0.14 -0.03,0.14
HELL  (via drill 0.6 pad 1.02)
  Top 0.4: v15.85,27.13 15.85,34.75 19.02,37.92 JP1.5
  Bottom 0.4: 7.59,20.14 8.86,20.14 v15.85,27.13
  Bottom 0.406: 7.59,20.14 7.59,8.71 BOARD2_LINKS.11
MPX_C  (via drill 0.6 pad 1.02)
  Top 0.406: IC9.8 43.69,2.9 v43.47,2.68
  Bottom 0.406: v43.47,2.68 37.44,2.68 36.17,1.41 7.59,1.41 5.05,3.95 5.05,6.17 BOARD2_LINKS.14
N$1
  Bottom 0.406: 15.85,55.7 15.85,49.35 83.16,49.35
N$2
  Top 0.406: 15.85,55.7 15.85,49.35 83.79,49.35
N$3  (via drill 0.6 pad 1.02)
  Top 0.406: IC8.10 58.39,8.71 v57.76,9.35 | v39.98,8.71 IC9.5 IC9.4
  Bottom 0.406: v57.76,9.35 40.61,9.35 v39.98,8.71
N$4  (via drill 0.6)
  Top 0.4: v28.57,6.62 28.57,7.42 26.57,7.42 IC7.11 | v62.17,6.62 61.77,7.02 61.77,7.42 60.37,7.42 IC8.9
  Bottom 0.4: v28.57,6.62 v62.17,6.62
N$5
  Bottom 0.4: IC1.8 29.18,22.68 30.45,21.41 45.06,21.41 IC2.11
N$6
  Top 0.4: IC3.11 59.57,22.82 56.81,25.59 56.81,41.42 50.8,47.42 44.77,47.42 44.77,41.22 41.21,37.66 41.21,25.26 38.77,22.82 IC2.8
N$7
  Bottom 0.406: IC3.8 54.9,22.68 56.17,21.41 68.87,21.41 70.14,22.68 IC4.11
N$8  (via drill 0.6 pad 1.02)
  Top 0.4: IC7.9 26.37,5.02 24.57,5.02 24.42,4.9
  Top 0.406: IC9.10 IC9.9 45.69,7.44 v46.33,8.08 | v24.1,7.76 24.1,5.22 24.42,4.9
  Bottom 0.406: v46.33,8.08 42.2,8.08 41.57,7.44 30.45,7.44 29.5,8.39 24.74,8.39 v24.1,7.76
N$11  (via drill 0.6 pad 1.02)
  Top 0.4: IC9.11 43.77,10.02 | IC7.13 26.57,10.02 28.77,10.02 v29.18,10.3
  Top 0.406: v29.18,10.3 28.87,9.98 | v40.61,12.21 40.61,11.89 42.52,9.98 IC9.11
  Bottom 0.406: v29.18,10.3 38.71,10.3 v40.61,12.21
N$16  (via drill 0.6)
  Top 0.4: v11.37,38.02 12.37,39.02 IC5.8 | IC6.1 6.57,30.42 6.57,33.22 v7.37,34.02
  Bottom 0.4: v7.37,34.02 v11.37,38.02
N$23
  Top 0.4: IC8.4 54.17,10.02 54.17,11.22 IC8.3
N$24
  Top 0.4: 41.53,7.44 41.53,1.02 53.24,1.02 56.17,3.95 56.17,7.13 55.85,7.44 IC8.6 53.97,7.42
  Top 0.406: 41.53,7.44 IC9.6
N$25  (via drill 0.6)
  Top 0.4: v13.37,16.42 9.37,20.42 9.37,29.22 9.97,29.82 9.97,41.62 10.02,41.62 10.02,42.82 12.37,42.82 IC5.11 | v41.97,15.22 41.97,13.42 42.77,12.62 43.57,12.62 IC9.13
  Bottom 0.4: v13.37,16.42 14.57,15.22 v41.97,15.22
NOT_GATE  (via drill 0.6)
  Top 0.4: v10.57,28.82 10.57,29.02 12.37,29.02 IC6.13 | v19.77,29.02 23.37,32.62 23.37,38.42 25.37,40.42 IC1.1 | v45.77,11.22 43.77,11.22 IC9.12 | v49.97,11.22 50.17,11.42 50.17,15.82 53.97,19.62 53.97,25.62 53.17,26.42 49.86,26.42 49.86,38.62 51.97,40.42 IC3.1
  Bottom 0.4: IC4.1 62.52,40.46 61.25,39.19 58.39,39.19 57.12,40.46 IC3.1 48.87,40.46 47.6,39.19 44.42,39.19 43.15,40.46 IC2.1 36.17,40.46 34.9,39.19 31.09,39.19 29.82,40.46 IC1.1 | v10.57,28.82 10.77,29.02 v19.77,29.02 | v49.97,11.22 v45.77,11.22
OPEN  (via drill 0.6)
  Top 0.4: v8.37,43.42 8.37,40.62 6.57,40.62 IC5.6 | v10.57,45.62 12.37,45.62 IC5.13
  Bottom 0.4: v8.37,43.42 v10.57,45.62
RS
  Bottom 0.4: BOARD2_RECHTS.2 81.25,8.08 JP2.7
SCAN  (via drill 0.6)
  Top 0.4: v32.77,3.94 32.97,4.14 32.97,20.02 IC1.10
  Bottom 0.4: 45.07,18.92 46.17,20.02 IC2.10 | 45.07,18.92 44.97,18.82 34.37,18.82 33.17,20.02 IC1.10 | 58.47,18.92 58.37,18.82 45.17,18.82 45.07,18.92 | 58.47,18.92 59.57,20.02 IC3.10 | IC4.10 72.17,20.02 70.97,18.82 58.57,18.82 58.47,18.92 | 29.18,3.94 v32.77,3.94
  Bottom 0.406: 29.18,3.94 16.16,3.94 15.85,3.63 12.99,3.63 12.67,3.95 12.67,6.17 BOARD2_LINKS.5
(copper drawn outside any net)
  shapes: Bottom circle x4

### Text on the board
Top: Component
Bottom: Print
